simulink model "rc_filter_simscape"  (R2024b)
settings: Solver=VariableStepAuto  StartTime=0.0  StopTime=10.0  RelTol=1e-3
libraries: fl_lib x6, nesl_utility x4, simulink x1

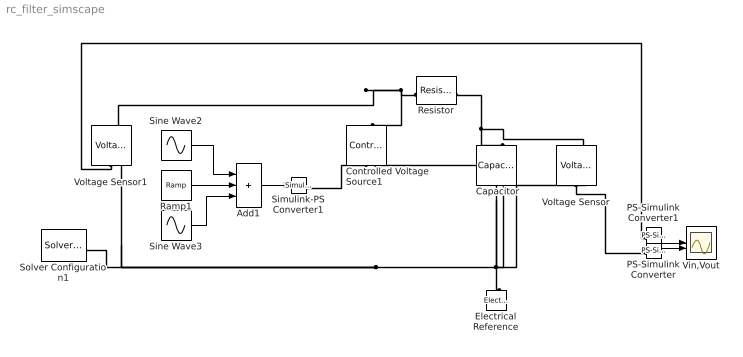
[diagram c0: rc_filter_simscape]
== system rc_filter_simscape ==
  Add1 : Sum  Inputs=+++
  Capacitor : fl_lib/Electrical/Electrical Elements/Capacitor  c=1e-3 F  r=1e-6 Ohm  g=0 1/Ohm  i_specify=off  i_priority=None  i=0 A  i_nominal_specify=off  i_nominal_value=1  i_nominal_unit=A  v_specify=off  v_priority=None  v=0 V  v_nominal_specify=off  v_nominal_value=1  v_nominal_unit=V  vc_specify=off  vc_priority=High  vc=0 V  vc_nominal_specify=off  vc_nominal_value=1  vc_nominal_unit=V
  Controlled Voltage Source1 : fl_lib/Electrical/Electrical Sources/Controlled Voltage Source
  Electrical Reference : fl_lib/Electrical/Electrical Elements/Electrical Reference
  PS-Simulink Converter : nesl_utility/PS-Simulink Converter  PhysicalDomain=network_engine_domain  SubClassName=ps_output  LeftPortType=input  RightPortType=output  PseudoPeriodic=off  Frequencies=[]  VectorFormat=inherit  Unit=inherit  AffineConversion=off
  PS-Simulink Converter1 : nesl_utility/PS-Simulink Converter  PhysicalDomain=network_engine_domain  SubClassName=ps_output  LeftPortType=input  RightPortType=output  PseudoPeriodic=off  Frequencies=[]  VectorFormat=inherit  Unit=inherit  AffineConversion=off
  Ramp1 : simulink/Sources/Ramp  slope=0.25  start=0  InitialOutput=0
  Resistor : fl_lib/Electrical/Electrical Elements/Resistor  R=100 Ohm  i_specify=off  i_priority=None  i=0 A  i_nominal_specify=off  i_nominal_value=1  i_nominal_unit=A  v_specify=off  v_priority=None  v=0 V  v_nominal_specify=off  v_nominal_value=1  v_nominal_unit=V
  Simulink-PS Converter1 : nesl_utility/Simulink-PS Converter  PhysicalDomain=network_engine_domain  SubClassName=ps_input  LeftPortType=input  RightPortType=output  PseudoPeriodic=off  Frequencies=[]  NoiseDistribution=none  NoiseParameters=[]  Unit=1  AffineConversion=off  FilteringAndDerivatives=provide  SimscapeFilterOrder=1  InputFilterTimeConstant=0.001  UdotUserProvided=0
  Sine Wave2 : Sin  Amplitude=2  Frequency=1.57  SampleTime=0
  Sine Wave3 : Sin  Amplitude=0.1  Frequency=31  SampleTime=0
  Solver Configuration1 : nesl_utility/Solver Configuration  PhysicalDomain=network_engine_domain  SubClassName=solver  LeftPortType=input  RightPortType=generic  Tones=[]  Harmonics=[]  SimulateNoise=off  Profile=off  UseLocalSampling=off  EnableSwitchedLinearOptims=on  FrequencyDomain=off  UseCCode=off  RelTol=0.001  AbsTol=0.001  MinStep=1e-09  ToWorkspace=off  RevertToSquareIcSolve=off  NumHomotopyIterations=100  PhasorMode=off  PhasorModeNumHarmonics=1  ConsistencySolver=NEWTON_XTOL_AFTER_FTOL  IndexReductionMethod=DerivativeReplacement  DoDC=off  ResidualTolerance=1e-09  ConsistencyTolSource=GLOBAL  ConsistencyAbsTol=0.001  ConsistencyRelTol=0.001  ConsistencyTolFactor=0.001  UseLocalSolver=off  LocalSolverChoice=NE_BACKWARD_EULER_ADVANCER  ResolveIndetEquations=on  FunctionEvalNumThread=1  LocalSolverSampleTime=0.001  DoFixedCost=off  MaxNonlinIter=3  MaxModeIter=2  ComputeImpulses=off  ImpulseIterations=2  LinearAlgebra=auto  LinearAlgebraNumThread=0  EquationFormulation=NE_TIME_EF  DelaysMemoryBudget=1024  AutomaticFiltering=on  FilteringTimeConstant=0.001  PartitionStorageMethod=AS_NEEDED  PartitionMemoryBudget=1024  PartitionMethod=ROBUST  MultibodyUseLocalSolver=off  MultibodyLocalSolverChoice=ODE1  MultibodyLocalSolverSampleTime=0.001
  Vin,Vout : Scope  NumInputPorts=2
  Voltage Sensor : fl_lib/Electrical/Electrical Sensors/Voltage Sensor
  Voltage Sensor1 : fl_lib/Electrical/Electrical Sensors/Voltage Sensor
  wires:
  PS-Simulink Converter1/1 -> Vin,Vout/1
  PS-Simulink Converter/1 -> Vin,Vout/2
  Ramp1/1 -> Add1/2
  Sine Wave2/1 -> Add1/1
  Sine Wave3/1 -> Add1/3
  Add1/1 -> Simulink-PS Converter1/1
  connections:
  Resistor/LConn1 -- Controlled Voltage Source1/LConn1 -- Voltage Sensor1/LConn1
  Voltage Sensor1/RConn2 -- Solver Configuration1/RConn1 -- Controlled Voltage Source1/RConn2 -- Electrical Reference/LConn1 -- Capacitor/RConn1 -- Voltage Sensor/RConn2
  Voltage Sensor/RConn1 -- PS-Simulink Converter/LConn1
  Resistor/RConn1 -- Voltage Sensor/LConn1 -- Capacitor/LConn1
  Voltage Sensor1/RConn1 -- PS-Simulink Converter1/LConn1
  Simulink-PS Converter1/RConn1 -- Controlled Voltage Source1/RConn1
